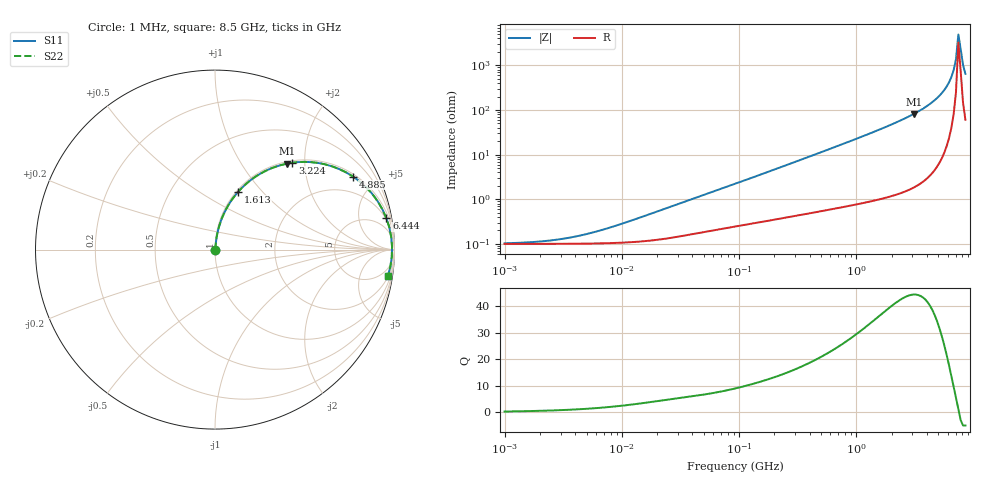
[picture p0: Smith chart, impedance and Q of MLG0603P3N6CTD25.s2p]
! S-Parameter Data Generated by TDK Corporation
! Copyright(C) 2025 TDK Corporation.
! All Rights Reserved.
! TDK P/N: MLG0603P3N6CTD25 (SMD / SMT Inductor (Coil))
! Property: L=3.6nH at 500MHz
! Size(LxWxT): 0.6x0.3x0.3mm
! Model Type: s2p (Touchstone File Format Version 1.0)
! Frequency: DC=Yes Start=1MHz Stop=8500MHz 198points Log-sweep
! Model Generated on Feb. 6, 2025
! Terms and conditions regarding TDK Simulation Models:
! 1)This simulation model is being provided solely for informational
!  purposes. Please refer to the specifications of the products in
!  terms of detailed characteristics of such products.
! 2)In no event shall TDK Corporation of any of its subsidiaries be
!  liable for any loss or damage arising, directly or indirectly,
!  from any information contained in this simulation model, including,
!  but not limited to loss or damages arising from any inaccuracies,
!  omissions or errors in connection with such information.
! 3)Any and all copyrights on this simulation model are owned by
!  TDK Corporation.  Duplication or redistribution of this simulation
!  model without prior written permission from TDK Corporation
!  is prohibited.
! 4)This simulation model is subject to any modification or change
!  without any prior notice.
! 5)Neither TDK Corporation nor any of its subsidiaries shall make any
!  warranty, express or implied, including but not limited to the
!  correctness, implied warranties of merchantability and fitness for
!  a particular purpose with respect to this simulation models.
! 6)The use of this simulation model shall be deemed to have consented
!  to the terms and conditions hereof.
! Port Assignments:
!  1 ---@@@--- 2
! Applicable Conditions:
!  Temperature = 25 degC
!  DC Bias Current = 0 A
!  Small Signal Operation
# Hz S MA R 50
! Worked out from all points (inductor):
!   197 points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, 1 MHz to 8.5 GHz, reference 50 ohm
!   read as one part in series: L = 4.15 nH near 12.67 MHz
!   highest Q = 44.5 at 3.079 GHz (marker M1), where L = 4.2 nH
!   self-resonance near 7.401 GHz
!   S11 on the Smith chart (normalised r, x): 1 MHz: 1.00, +0.00; 1.613 GHz: 1.02, +0.75; 3.224 GHz: 1.04, +1.74; 4.885 GHz: 1.11, +3.71; 6.444 GHz: 2, +11; 8.5 GHz: 2, -13
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1000000  0.001034 14.8  0.999 -0.0  0.999 -0.0  0.001034 14.8
2295435  0.001171 31.1  0.999 -0.0  0.999 -0.0  0.001171 31.1
4587603  0.001577 49.9  0.999 -0.1  0.999 -0.1  0.001577 49.9
8360083  0.002432 64.4  0.999 -0.1  0.999 -0.1  0.002432 64.4
2.10461e7  0.005578 76.7  0.9987 -0.3  0.9987 -0.3  0.005578 76.7
9.219544e7  0.02209 82.4  0.9973 -1.3  0.9973 -1.3  0.02209 82.4
4.229561e8  0.09515 81.6  0.9905 -5.5  0.9905 -5.5  0.09515 81.6
9.270694e8  0.2037 76.2  0.9719 -11.7  0.9719 -11.7  0.2037 76.2
1.613203e9  0.3469 68.2  0.9285 -20.3  0.9285 -20.3  0.3469 68.2
1.940355e9  0.4128 64.2  0.9005 -24.4  0.9005 -24.4  0.4128 64.2
3.07866e9  0.6239 50.1  0.7676 -38.6  0.7676 -38.6  0.6239 50.1
3.224109e9  0.6483 48.3  0.7469 -40.4  0.7469 -40.4  0.6483 48.3
4.061159e9  0.7741 37.9  0.6147 -50.7  0.6147 -50.7  0.7741 37.9
4.884749e9  0.87 27.9  0.4683 -60.4  0.4683 -60.4  0.87 27.9
5.610304e9  0.9298 19.5  0.3333 -68.3  0.3333 -68.3  0.9298 19.5
6.152938e9  0.9596 13.4  0.2329 -73.4  0.2329 -73.4  0.9596 13.4
6.44363e9  0.9707 10.4  0.1802 -75.5  0.1802 -75.5  0.9707 10.4
6.748056e9  0.979 7.2  0.1263 -76.9  0.1263 -76.9  0.979 7.2
7.066863e9  0.9844 4.0  0.07183 -75.4  0.07183 -75.4  0.9844 4.0
7.400733e9  0.9866 0.9  0.02013 -47.8  0.02013 -47.8  0.9866 0.9
8.116539e9  0.9816 -5.5  0.0968 76.3  0.0968 76.3  0.9816 -5.5
8.5e9  0.9745 -8.7  0.1511 76.0  0.1511 76.0  0.9745 -8.7
